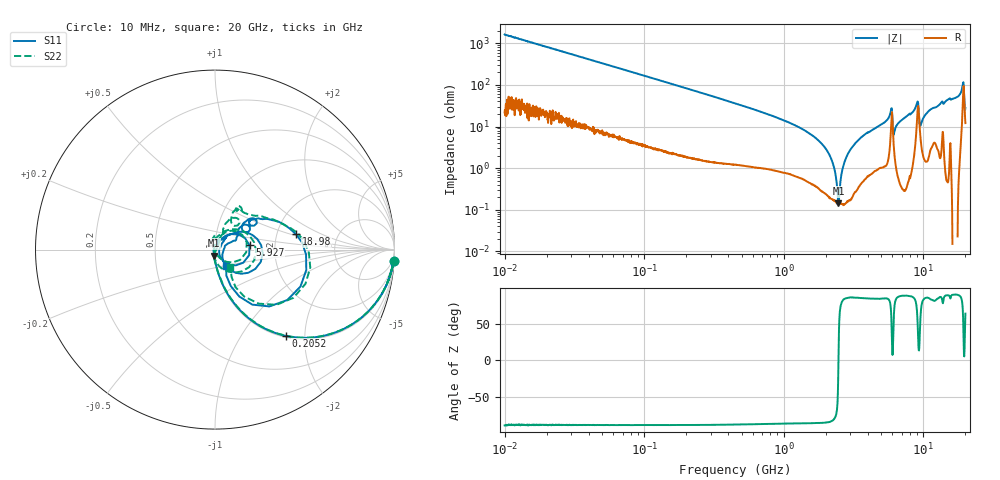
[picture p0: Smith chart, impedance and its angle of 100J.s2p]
!Keysight Technologies,P5008B,MY61100088,A.16.20.02
!Date: Monday, November 06, 2023 16:19:37
!Correction: S11(C  2-Port  )
!S21(C  2-Port  )
!S12(C  2-Port  )
!S22(C  2-Port  )
!S2P File: Measurements: S11, S21, S12, S22:Log Frequency Sweep
# Hz S  dB  R 50
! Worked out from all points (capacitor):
!   1601 points, 10 MHz to 20 GHz, reference 50 ohm
!   read as one part in series: C = 9.79 pF near 10.39 MHz
!   lowest |Z| = 142 mohm at 2.461 GHz (marker M1)
!   series resonance near 2.465 GHz, so ESL is about 430 pH
!   S11 on the Smith chart (normalised r, x): 10 MHz: 1, -32; 205.2 MHz: 1.03, -1.62; 5.927 GHz: 1.47, +0.07; 18.98 GHz: 2.56, +0.55; 20 GHz: 1.11, -0.21
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1e7  -0.02 -3.5  -24.25 85.7  -24.26 85.7  -0.02 -3.5
3.555162e7  -0.23 -12.1  -13.60 76.6  -13.60 76.6  -0.24 -12.1
1.263918e8  -2.06 -36.9  -4.45 51.9  -4.45 51.9  -2.07 -37.0
2.051915e8  -4.10 -50.5  -2.28 38.2  -2.29 38.2  -4.13 -50.5
4.472136e8  -9.25 -68.8  -0.65 19.4  -0.65 19.4  -9.41 -68.9
1.589917e9  -21.26 -86.4  -0.10 2.4  -0.10 2.4  -22.39 -89.0
2.461408e9  -29.53 -96.8  -0.06 -1.9  -0.06 -1.9  -29.55 -100.9
3.211587e9  -42.00 -174.2  -0.07 -4.7  -0.07 -4.7  -38.36 -84.6
3.599441e9  -37.08 107.2  -0.07 -6.0  -0.08 -6.0  -44.55 -15.5
5.652411e9  -22.39 57.1  -0.18 -14.3  -0.19 -14.3  -21.51 66.2
5.927413e9  -14.25 7.1  -1.66 -15.0  -1.66 -15.0  -14.82 13.2
6.245393e9  -28.81 -47.1  -0.16 -10.3  -0.16 -10.3  -42.06 -88.7
6.425969e9  -32.54 -13.6  -0.09 -11.8  -0.10 -11.8  -35.74 119.2
6.867879e9  -29.16 26.0  -0.06 -14.1  -0.07 -14.1  -28.06 114.2
9.08967e9  -11.76 5.6  -1.99 -25.5  -2.00 -25.5  -13.09 10.7
9.441767e9  -17.44 -54.0  -0.71 -13.6  -0.71 -13.6  -19.38 -71.7
9.901129e9  -25.53 -39.4  -0.16 -18.7  -0.16 -18.6  -33.45 -107.4
1.018741e10  -26.54 -13.2  -0.11 -20.5  -0.11 -20.5  -40.24 119.3
1.147208e10  -19.64 25.1  -0.29 -25.9  -0.29 -25.9  -21.18 64.0
1.653881e10  -12.12 39.5  -0.33 -41.9  -0.34 -41.8  -11.79 59.8
1.898171e10  -6.74 10.7  -2.55 -63.1  -2.55 -63.1  -6.55 11.2
2e10  -19.03 -56.2  -1.14 -33.3  -1.14 -33.2  -17.77 -49.3
